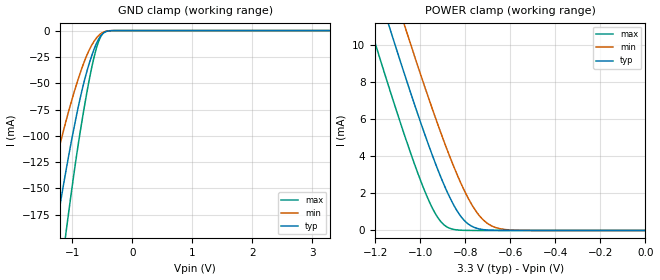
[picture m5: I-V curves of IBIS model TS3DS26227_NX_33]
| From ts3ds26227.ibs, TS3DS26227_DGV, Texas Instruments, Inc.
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[Model]   TS3DS26227_NX_33
Model_type  Terminator
| variable   typ   min   max
C_comp   2.57pF   2.27pF   2.97pF
| C_tri-state   2.57pF   2.27pF   2.97pF
[Temperature Range]   40   100   -40
| Ambient temperature   25   85   -40
[Voltage range]   3.3   3   3.6
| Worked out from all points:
|   GND clamp passes 1 mA (typ) near -0.44 V on its own axis
|   POWER clamp passes 1 mA (typ) near -0.83 V on its own axis
[GND Clamp]
| TS3DS26227_NX_33
|   Voltage   I(typ)   I(min)   I(max)
-3.3V     -1.037A    -774.5mA   -1.262A
-1.565V   -297.4mA   -199.7mA   -405.6mA
-1.515V   -278.4mA   -186.2mA   -381.7mA
-1.29V    -196mA     -128.7mA   -276.2mA
-1.265V   -187.3mA   -122.7mA   -264.7mA
-1.105V   -133.8mA   -86.44mA   -193mA
-895mV    -71.68mA   -45.27mA   -106.7mA
-725mV    -32.95mA   -19.55mA   -49.57mA
-590mV    -11.55mA   -6.683mA   -15.56mA
-485mV    -2.582mA   -1.612mA   -2.556mA
-320mV    -48.3uA    -47.75uA   -17.69uA
3.3V      4.818nA    15.45nA    373.6pA
[POWER Clamp]
| TS3DS26227_NX_33
|   Voltage   I(typ)   I(min)   I(max)
-3.3V     101.2mA    103.7mA    98.32mA
-1.215V   14.04mA    16.7mA     10.7mA
-1.13V    10.72mA    13.38mA    7.394mA
-1.07V    8.447mA    11.09mA    5.157mA
-1.06V    8.074mA    10.71mA    4.796mA
-980mV    5.197mA    7.759mA    2.13mA
-910mV    2.924mA    5.324mA    501.7uA
-815mV    691.1uA    2.434mA    11.72uA
-760mV    165.2uA    1.179mA    1.002uA
-715mV    40.41uA    514.1uA    133.5nA
-600mV    895.3nA    27.97uA    1.516nA
-48.03fV  4.818nA    8.743nA    473pA
